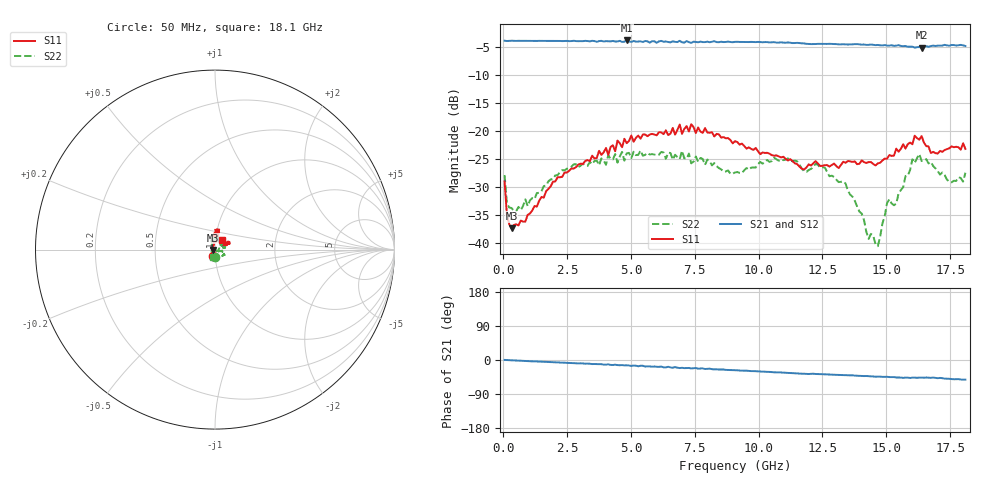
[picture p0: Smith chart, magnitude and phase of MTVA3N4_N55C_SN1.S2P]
! Network Analyzer HP8720D.06.14 Serial No. US36140669
! 27 Jun 2005  09:26:30
! Frequency  S11  S21  S12  S22
# HZ  S  DB R 50
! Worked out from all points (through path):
!   201 points, 50 MHz to 18.1 GHz, reference 50 ohm
!   highest |S21| = -3.79 dB at 4.833 GHz (marker M1); lowest = -5.1 dB at 16.39 GHz (marker M2)
!   group delay of S21, straight-line fit = 8.09 ps
!   lowest |S11| = -37.5 dB at 320.8 MHz (marker M3), VSWR 1.03, Z = 48.7 - j0.262 ohm
!   |S11| at or under -10 dB: start of sweep to end of sweep
!   |S22| runs from -40.6 to -23.5 dB; largest |S21 - S12| = 0.019
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5e7  -29.04 -103.9  -3.83 0.2  -3.87 0.3  -27.88 -91.9
1.4025e8  -35.04 -131.4  -3.89 -0.2  -3.88 -0.2  -32.93 -142.0
3.2075e8  -37.45 -168.4  -3.84 -0.7  -3.86 -0.7  -33.78 -169.6
2.12575e9  -28.27 96.5  -3.88 -6.5  -3.89 -6.3  -27.90 113.2
3.1185e9  -25.90 90.6  -3.92 -9.0  -3.94 -9.3  -25.85 112.9
4.83325e9  -22.18 86.3  -3.79 -14.0  -3.90 -14.7  -23.99 91.9
6.09675e9  -20.22 81.7  -3.95 -18.1  -3.90 -18.0  -24.24 83.6
6.99925e9  -20.50 83.9  -4.11 -20.6  -4.16 -21.6  -23.55 72.0
7.36025e9  -18.80 78.1  -4.22 -22.3  -4.08 -21.7  -25.78 72.9
9.075e9  -21.82 93.4  -4.04 -26.9  -4.03 -27.1  -27.42 31.6
1.060925e10  -24.42 86.6  -4.09 -32.5  -4.15 -32.6  -24.78 11.1
1.21435e10  -25.76 74.8  -4.43 -36.3  -4.40 -36.6  -26.43 39.7
1.3407e10  -25.68 48.6  -4.50 -39.9  -4.47 -40.1  -29.40 33.6
1.43095e10  -25.56 23.4  -4.58 -42.8  -4.53 -42.9  -39.31 -45.9
1.46705e10  -25.80 22.2  -4.59 -44.0  -4.60 -44.0  -40.62 -39.3
1.512175e10  -24.30 21.4  -4.71 -45.1  -4.63 -45.0  -32.22 -25.7
1.53925e10  -23.16 23.2  -4.71 -46.1  -4.62 -45.8  -32.99 -24.9
1.602425e10  -22.37 28.2  -4.90 -46.6  -5.07 -47.7  -25.06 -15.1
1.638525e10  -20.90 22.6  -5.08 -46.3  -4.87 -46.5  -25.38 -33.6
1.674625e10  -23.94 29.9  -4.79 -47.1  -4.94 -47.1  -25.52 -49.9
1.75585e10  -22.75 54.4  -4.61 -50.3  -4.63 -51.0  -29.19 -78.6
1.81e10  -23.20 53.1  -4.78 -51.8  -4.76 -52.7  -27.47 -106.3
